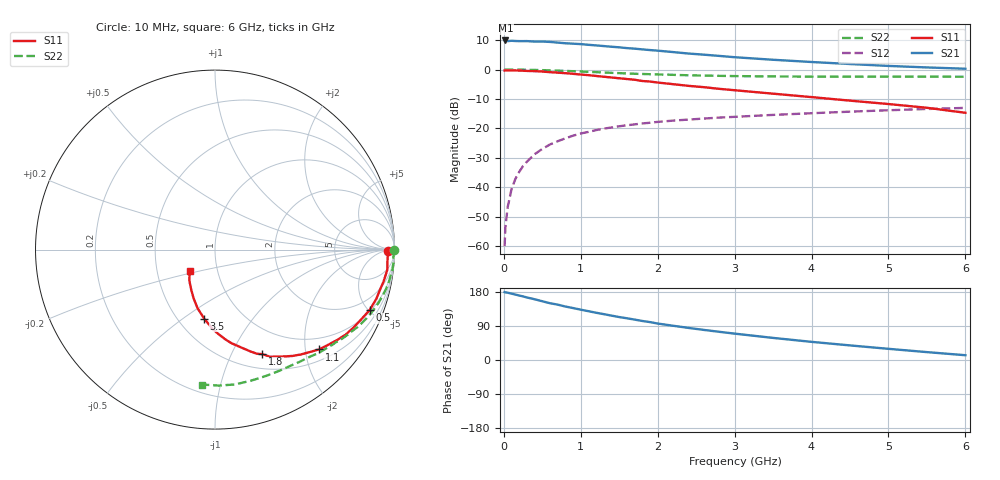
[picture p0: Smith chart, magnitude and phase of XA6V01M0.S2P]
! SIEMENS Discrete & RF Semiconductors
! BFY180
! Si NPN RF Bipolar Junction Transistor in MICRO-X
! VCE = 6 V  IC = 1 mA
! Common Emitter S-Parameters:  May  1997
# GHz  S  MA  R  50
!  f  S11  S21  S12  S22
! GHz  MAG  ANG  MAG  ANG  MAG  ANG  MAG  ANG
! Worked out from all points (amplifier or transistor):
!   36 points, 10 MHz to 6 GHz, reference 50 ohm
!   highest |S21| = 9.9 dB at 20 MHz (marker M1)
!   |S21| within 3 dB of that: start of sweep to 1.787 GHz
!   unconditionally stable (mu >= 1): 4.153 GHz to end of sweep
!   at 250 MHz: K = 0.09, MSG = 21.2 dB, |S12| = -32.8 dB
!   at 1.4 GHz: K = 0.49, MSG = 13.7 dB, |S12| = -19.7 dB
!   at 6 GHz: K = 1.05, MAG = 5.3 dB, |S12| = -13.0 dB
!   S11 on the Smith chart (normalised r, x): 10 MHz: 53, -10; 500 MHz: 1.09, -5.07; 1.1 GHz: 0.73, -2.29; 1.8 GHz: 0.67, -1.32; 3.5 GHz: 0.67, -0.60; 6 GHz: 0.73, -0.18
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0.01  0.9639 -0.4  3.088 179.1  0.001 92.4  0.9967 -0.2
0.02  0.9633 -0.9  3.122 178.5  0.0021 93.5  0.9999 -0.6
0.05  0.9633 -2.0  3.043 177.6  0.0046 89.8  0.9971 -1.3
0.1  0.9632 -4.3  3.082 175.1  0.0093 88.0  0.9943 -2.6
0.15  0.9665 -6.7  3.055 172.7  0.0139 86.4  0.9976 -3.9
0.3  0.9483 -12.9  3.044 165.0  0.0272 81.7  0.99 -7.9
0.5  0.9248 -21.4  2.992 155.0  0.0449 74.9  0.9778 -13.0
0.6  0.9037 -25.3  2.948 149.8  0.0534 72.5  0.9683 -15.4
0.8  0.8683 -33.1  2.797 141.1  0.0679 66.7  0.9481 -20.1
1  0.8234 -40.2  2.706 132.8  0.082 61.4  0.9263 -24.5
1.1  0.8033 -43.8  2.633 128.8  0.0874 59.5  0.915 -26.5
1.5  0.7114 -56.8  2.386 113.3  0.1087 51.0  0.8695 -34.2
1.8  0.6395 -65.6  2.202 103.0  0.1216 46.5  0.8418 -39.1
2  0.6019 -70.7  2.095 96.2  0.1291 43.6  0.8266 -42.2
2.2  0.5647 -75.0  1.982 90.4  0.1358 40.7  0.8139 -45.2
2.4  0.5291 -80.1  1.872 84.7  0.1414 38.4  0.7993 -48.0
2.8  0.4707 -87.7  1.706 74.4  0.1528 34.4  0.7825 -53.2
3.5  0.3893 -98.9  1.467 58.3  0.1698 28.2  0.7644 -62.1
4  0.3406 -106.6  1.344 47.9  0.1813 24.1  0.7588 -68.4
4.5  0.2965 -113.7  1.242 38.5  0.1927 20.3  0.7574 -74.9
5.5  0.2243 -129.6  1.087 20.8  0.214 12.4  0.7579 -88.5
6  0.1844 -140.0  1.033 12.6  0.2234 8.2  0.7551 -95.4
